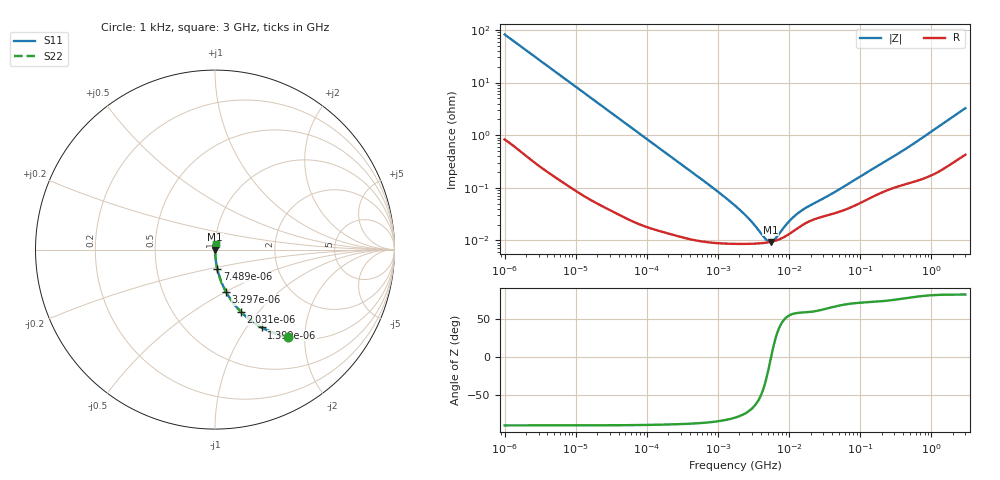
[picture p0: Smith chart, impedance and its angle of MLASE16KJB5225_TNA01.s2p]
! MLASE16KJB5225_TNA01  S-PARAMETER MODEL  ( Standard Model )
! Model Generated by TAIYO YUDEN Corporation (http://www.ty-top.com)
! Version 1.0
! TAIYO YUDEN Control No. 220601
! Copyright(c) 2012 TAIYO YUDEN CO.,LTD. All Rights Reserved.
! Product Description (link to TY-COMPAS)
! https://ds.yuden.co.jp/TYCOMPAS/or/detail?pn=MLASE16KJB5225KTNA01&u=M
! Products Name : Multilayer Ceramic Capacitors
! Characteristics :
!  Capacitance : 2.2 [uF] , Rated Voltage : 16 [V] , TCC : X5R
!  Case Size : 1.6 x 0.8 / 0.063 x 0.031 [mm/inch] , Thickness : 0.45 / 0.018 [mm/inch]
!  (Conditions: Temperature = 25 [degC] , DC Bias Voltage = 0 [V])
! External Node Assignments :
!  1  o---| |---o  2
! GND o---------o GND
! Frequency Range : 1kHz  -  3GHz  [ 401 STEP ]
# MHZ S RI R 50
! Freq[MHz].  S11 Real  S11 Imag  S21 Real  S21 Imag  S12 Real  S12 Imag  S22 Real  S22 Imag
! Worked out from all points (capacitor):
!   401 points, 1 kHz to 3 GHz, reference 50 ohm
!   read as one part in series: C = 1.93 uF near 1.077 kHz
!   lowest |Z| = 9.35 mohm at 5.502 MHz (marker M1)
!   series resonance near 5.559 MHz, so ESL is about 420 pH
!   S11 on the Smith chart (normalised r, x): 1 kHz: 1.02, -1.64; 1.399 kHz: 1.01, -1.18; 2.031 kHz: 1.01, -0.81; 3.297 kHz: 1.00, -0.50; 7.489 kHz: 1.00, -0.22; 3 GHz: 1.01, +0.06
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0.001  0.4041 -0.4857  0.5959 0.4857  0.5959 0.4857  0.4041 -0.4857
0.001399  0.2598 -0.4335  0.7402 0.4335  0.7402 0.4335  0.2598 -0.4335
0.002031  0.1444 -0.3467  0.8556 0.3467  0.8556 0.3467  0.1444 -0.3467
0.003297  0.0614 -0.2353  0.9386 0.2353  0.9386 0.2353  0.0614 -0.2353
0.007489  0.0133 -0.1095  0.9867 0.1095  0.9867 0.1095  0.0133 -0.1095
0.01216  0.00541 -0.0682  0.9946 0.0682  0.9946 0.0682  0.00541 -0.0682
0.033275  0.000987 -0.0252  0.999 0.0252  0.999 0.0252  0.000987 -0.0252
0.147855  0.000184 -0.00574  0.9998 0.00574  0.9998 0.00574  0.000184 -0.00574
0.762639  9.23e-05 -0.00111  0.9999 0.00111  0.9999 0.00111  9.23e-05 -0.00111
1.732051  8.58e-05 -0.00045  0.9999 0.00045  0.9999 0.00045  8.58e-05 -0.00045
2.812335  8.59e-05 -0.000229  0.9999 0.000229  0.9999 0.000229  8.59e-05 -0.000229
4.566395  8.96e-05 -6.21e-05  0.9999 6.21e-05  0.9999 6.21e-05  8.96e-05 -6.21e-05
4.919932  9.09e-05 -3.84e-05  0.9999 3.84e-05  0.9999 3.84e-05  9.09e-05 -3.84e-05
5.502215  9.34e-05 -3.18e-06  0.9999 3.18e-06  0.9999 3.18e-06  9.34e-05 -3.18e-06
6.387174  9.84e-05 4.39e-05  0.9999 -4.39e-05  0.9999 -4.39e-05  9.84e-05 4.39e-05
9.273352  0.000124 0.000164  0.9999 -0.000164  0.9999 -0.000164  0.000124 0.000164
12.03889  0.000157 0.000249  0.9998 -0.000249  0.9998 -0.000249  0.000157 0.000249
15.62917  0.000198 0.000329  0.9998 -0.000329  0.9998 -0.000329  0.000198 0.000329
21.06097  0.000243 0.000419  0.9998 -0.000419  0.9998 -0.000419  0.000243 0.000419
44.39505  0.00033 0.000771  0.9997 -0.000771  0.9997 -0.000771  0.00033 0.000771
256.0921  0.000938 0.0034  0.9991 -0.0034  0.9991 -0.0034  0.000938 0.0034
3000  0.00525 0.032  0.9947 -0.032  0.9947 -0.032  0.00525 0.032
